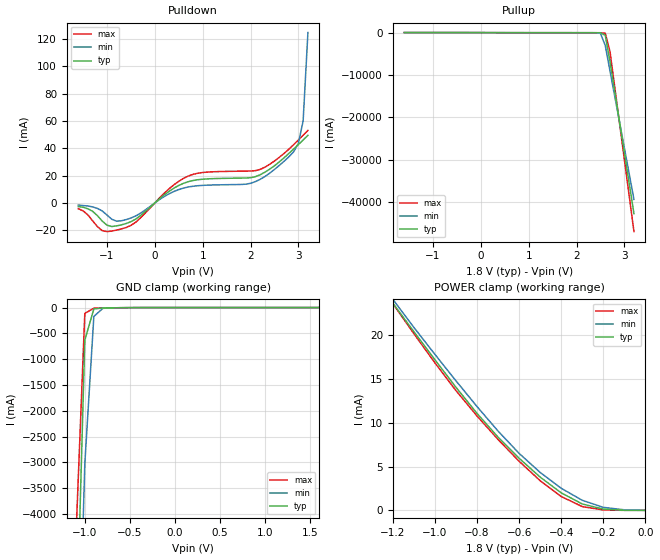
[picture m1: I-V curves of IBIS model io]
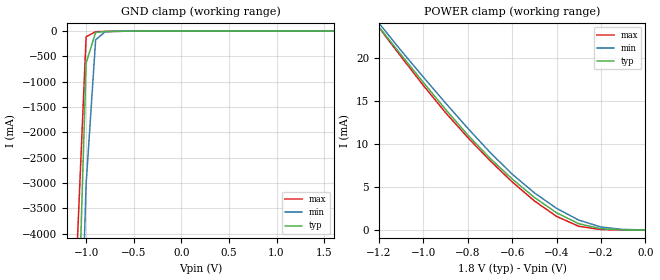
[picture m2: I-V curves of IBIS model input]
[IBIS Ver]	2.1
[File Name]	63r918a.ibs
[File Rev]	1.1
[Date]	8/31/99
[Source]	File originated at Motorola
[Notes]	This file is valid for:  MCM63R918A
|		(the 8M Late Write HSTL FSRAM).
|		BEWARE! This model has been generated with the
|		HSTL programmed to 50 impedance. The HSTL is capable
|		of impedances from 35ohms to 70 ohms.  This device is
|		internally regulated.  Model assumes a vddq = 1.5V
|		and a vref = 0.75V.
[Disclaimer]This information is for modeling purposes only and
|		is not guaranteed.
[Component]		512Kx18FSRAM
[Manufacturer]	Motorola
[Package]
|  RLC Data is subject to change after further study of package
|		typ		min		max
R_pkg		100m		NA		NA
L_pkg		5nH		NA		NA
C_pkg		1.5pF		NA		NA
[Pin]		signal_name	model_name	R_pin		L_pin		C_pin
1A		VDDQ		POWER		NA		NA		NA
1B		NC		NC		NA		NA		NA
1C		NC		NC		NA		NA		NA
1D		DQb		io		NA		NA		NA
1E		NC		NC		NA		NA		NA
1F		VDDQ		POWER		NA		NA		NA
1G		NC		NC		NA		NA		NA
1H		DQb		io		NA		NA		NA
1J		VDDQ		POWER		NA		NA		NA
1K		NC		NC		NA		NA		NA
1L		DQb		io		NA		NA		NA
1M		VDDQ		POWER		NA		NA		NA
1N		DQb		io		NA		NA		NA
1P		NC		NC		NA		NA		NA
1R		NC		NC		NA		NA		NA
1T		NC		NC		NA		NA		NA
1U		VDDQ		POWER		NA		NA		NA
2A		SA		input		NA		NA		NA
2B		NC	 	NC		NA		NA		NA
2C		SA		input		NA		NA		NA
2D		NC		NC		NA		NA		NA
2E		DQb		io		NA		NA		NA
2F		NC		NC		NA		NA		NA
2G		DQb		io		NA		NA		NA
2H		NC		NC		NA		NA		NA
2J		VDD		POWER		NA		NA		NA
2K		DQb		io		NA		NA		NA
2L		NC		NC		NA		NA		NA
2M		DQb		io		NA		NA		NA
2N		NC		NC		NA		NA		NA
2P		DQb		io		NA		NA		NA
2R		SA		input		NA		NA		NA
2T		SA		input		NA		NA		NA
2U		TMS		input		NA		NA		NA
3A		SA		input		NA		NA		NA
3B		SA		input		NA		NA		NA
3C		SA		input		NA		NA		NA
3D		VSS		GND		NA		NA		NA
3E		VSS		GND		NA		NA		NA
3F		VSS		GND		NA		NA		NA
3G		SBb#		input		NA		NA		NA
3H		VSS		GND		NA		NA		NA
3J		Vref		POWER		NA		NA		NA
3K		VSS		GND		NA		NA		NA
3L		VSS		GND		NA		NA		NA
3M		VSS		GND		NA		NA		NA
3N		VSS		GND		NA		NA		NA
3P		VSS		GND		NA		NA		NA
3R		VSS		GND		NA		NA		NA
3T		SA		input		NA		NA		NA
3U		TDI		input		NA		NA		NA
4A		NC		NC		NA		NA		NA
4B		NC		NC		NA		NA		NA
4C		VDD		POWER		NA		NA		NA
4D		ZQ		input		NA		NA		NA
4E		SS#		input		NA		NA		NA
4F		G#		input		NA		NA		NA
4G		NC		NC		NA		NA		NA
4H		NC		NC		NA		NA		NA
4J		VDD		POWER		NA		NA		NA
4K		CK		input		NA		NA		NA
4L		CK#		input		NA		NA		NA
4M		SW#		input		NA		NA		NA
4N		SA		input		NA		NA		NA
4P		SA		input		NA		NA		NA
4R		VDD		POWER		NA		NA		NA
4T		NC		NC		NA		NA		NA
4U		TCK		input		NA		NA		NA
5A		SA		input		NA		NA		NA
5B		SA		input		NA		NA		NA
5C		SA		input		NA		NA		NA
5D		VSS		GND		NA		NA		NA
5E		VSS		GND		NA		NA		NA
5F		VSS		GND		NA		NA		NA
5G		VSS		GND		NA		NA		NA
5H		VSS		GND		NA		NA		NA
5J		Vref		POWER		NA		NA		NA
5K		VSS		GND		NA		NA		NA
5L		SBa#		input		NA		NA		NA
5M		VSS		GND		NA		NA		NA
5N		VSS		GND		NA		NA		NA
5P		VSS		GND		NA		NA		NA
5R		VDD		POWER		NA		NA		NA
5T		SA		input		NA		NA		NA
5U		TDO		input		NA		NA		NA
6A		SA		input		NA		NA		NA
6B		SA		input		NA		NA		NA
6C		SA		input		NA		NA		NA
6D		DQa		io		NA		NA		NA
6E		NC		NC		NA		NA		NA
6F		DQa		io		NA		NA		NA
6G		NC		NC		NA		NA		NA
6H		DQa		io		NA		NA		NA
6J		VDD		POWER		NA		NA		NA
6K		NC		NC		NA		NA		NA
6L		DQa		io		NA		NA		NA
6M		NC		NC		NA		NA		NA
6N		DQa		io		NA		NA		NA
6P		NC		NC		NA		NA		NA
6R		SA		input		NA		NA		NA
6T		SA		input		NA		NA		NA
6U		NC		NC		NA		NA		NA
7A		VDDQ		POWER		NA		NA		NA
7B		NC		NC		NA		NA		NA
7C		NC		NC		NA		NA		NA
7D		NC		NC		NA		NA		NA
7E		DQa		io		NA		NA		NA
7F		VDDQ		POWER		NA		NA		NA
7G		DQa		io		NA		NA		NA
7H		NC		NC		NA		NA		NA
7J		VDDQ		POWER		NA		NA		NA
7K		DQa		io		NA		NA		NA
7L		NC		NC		NA		NA		NA
7M		VDDQ		POWER		NA		NA		NA
7N		NC		NC		NA		NA		NA
7P		DQa		io		NA		NA		NA
7R		NC		NC		NA		NA		NA
7T		ZZ		input		NA		NA		NA
7U		VDDQ		POWER		NA		NA		NA
| Models and submodels in the file (2): io (I/O), input (Input)
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[Model]	io
Model_type	I/O
Polarity	Non-Inverting
Enable	Active-Low
|		signals  DQa, DQb, DQc, DQd
|		typ		min		max
C_comp	6pF		5pF		8pF
|   |   |\ |   Rref
|   |Driver| \|------o----/\/\/\----o Vref
|   |   | /|   |
|   |   |/ |   === Cref
|   GND
Cref = 20pF
Rref = 50
Vref = 0.75
Vmeas = 0.75
Vinl = 0.55
Vinh = 0.95
|			typ		min		max
[Voltage range]	1.8V		1.6V		2.0V
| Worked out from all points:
|   slope of the pulldown table from 0 to 0.27 V, typ, clamps not added: 34.6 ohm
|   slope of the pullup table from 0 to 0.27 V, typ, clamps not added: 38.3 ohm
|   GND clamp passes 1 mA (typ) near -0.46 V on its own axis
|   POWER clamp passes 1 mA (typ) near -0.32 V on its own axis
| Temperature   50 C		110 C		0 C
[Pullup]
|	Voltage  	I(typ)   I(min)   I(max)
-1.6V     21.24mA    20.2mA     22.31mA
2.4V      -22.72mA   -29.33mA   -23.05mA
2.5V      -41.32mA   -183.8mA   -26.71mA
2.6V      -643.3mA   -3.031A    -127.5mA
2.7V      -6.854A    -9.094A    -4.526A
3.2V      -42.8A     -39.42A    -47.05A
[Pulldown]
|	Voltage  	I(typ)   I(min)   I(max)
-1.6V     -2.6mA     -1.5mA     -4.2mA
-1.3V     -6.1mA     -2.9mA     -13.1mA
-1.1V     -13.23mA   -5.83mA    -20.28mA
-800mV    -16.83mA   -13.33mA   -19.9mA
-400mV    -11.84mA   -9.526mA   -14.14mA
300mV     8.588mA    6.744mA    10.42mA
700mV     15.59mA    11.7mA     19.72mA
1.9V      18.28mA    13.75mA    23.33mA
2.4V      24.74mA    21.78mA    28.31mA
3V        42.77mA    43.53mA    46.09mA
3.1V      46.11mA    60.17mA    49.58mA
3.2V      49.54mA    124.9mA    53.11mA
|   TRI-STATED OUTPUT
|   typ		min		max
|Voltage range	1.8V		1.6V		2.0V
| Temperature   50 C		110 C		0 C
|****************  FOR OUTPUTS  *********
[GND_clamp]
|	Voltage  	I(typ)   I(min)   I(max)
-1.6V     -42.8A     -39.42A    -47.05A
-1.1V     -6.845A    -9.088A    -4.513A
-1V       -630.6mA   -3.023A    -113mA
-900mV    -26.86mA   -171.7mA   -11.77mA
-800mV    -7.649mA   -14.96mA   -7.659mA
-400mV    -426.2uA   -590.8uA   -289.2uA
1.6V      503.2nA    5.232uA    33.56nA
[POWER_clamp]
|	Voltage  	I(typ)   I(min)   I(max)
-1.6V     36.82mA    115mA      37.45mA
-1.2V     23.66mA    24.1mA     23.6mA
-1.1V     20.4mA     20.89mA    20.18mA
-900mV    14.05mA    14.79mA    13.67mA
-800mV    11.07mA    11.85mA    10.77mA
-700mV    8.36mA     9.05mA     8.091mA
-600mV    5.943mA    6.505mA    5.602mA
-500mV    3.794mA    4.326mA    3.384mA
-400mV    1.998mA    2.519mA    1.582mA
-300mV    726.9uA    1.148mA    428.5uA
-200mV    140.6uA    343.6uA    46.31uA
0V        503.2nA    5.232uA    33.56nA
[Ramp]
| 		typ			min			max
|Temperature  50 C		110 C			0 C
dV/dt_r	0.436/0.086n	0.422/0.103n	0.451/0.076n
dV/dt_f	0.489/0.103n	0.392/0.124n	0.557/0.079n
[Model]		input
Model_type		Input
Polarity		Non-Inverting
| signals  SA, G#,  SS#, SBa#, SBb#, SBc#, SBd#, CK#, CK,
|   TDI,  TMS,  TCK, SW#, ZQ, TDO
|  	* TDO has been listed here, but it is technically an output pin.
| 	This simplification has been made under the assumption
|  	that its structure is similar to the input pin's structure.
Vinl = 0.65V
Vinh = 0.85V
|			typ		min		max
C_comp		5pF		4pF		5pF
|			typ		min		max
[Voltage range]	1.8V		1.6V		2.0V
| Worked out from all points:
|   GND clamp passes 1 mA (typ) near -0.46 V on its own axis
|   POWER clamp passes 1 mA (typ) near -0.32 V on its own axis
| Temperature   50 C		110 C		0 C
[GND_clamp]
|	Voltage  	I(typ)   I(min)   I(max)
-1.6V     -42.8A     -39.42A    -47.05A
-1.1V     -6.845A    -9.088A    -4.513A
-1V       -630.6mA   -3.023A    -113mA
-900mV    -26.86mA   -171.7mA   -11.77mA
-800mV    -7.649mA   -14.96mA   -7.659mA
-400mV    -426.2uA   -590.8uA   -289.2uA
1.6V      503.2nA    5.232uA    33.56nA
[POWER_clamp]
|	Voltage	I(typ)		I(min)		I(max)
-1.6V     36.82mA    115mA      37.45mA
-1.2V     23.66mA    24.1mA     23.6mA
-1.1V     20.4mA     20.89mA    20.18mA
-900mV    14.05mA    14.79mA    13.67mA
-800mV    11.07mA    11.85mA    10.77mA
-700mV    8.36mA     9.05mA     8.091mA
-600mV    5.943mA    6.505mA    5.602mA
-500mV    3.794mA    4.326mA    3.384mA
-400mV    1.998mA    2.519mA    1.582mA
-300mV    726.9uA    1.148mA    428.5uA
-200mV    140.6uA    343.6uA    46.31uA
0V        503.2nA    5.232uA    33.56nA
